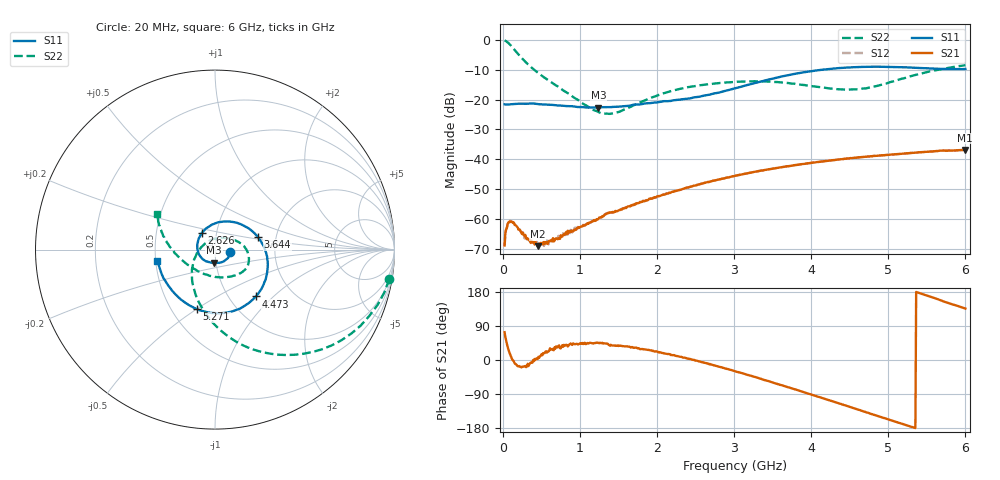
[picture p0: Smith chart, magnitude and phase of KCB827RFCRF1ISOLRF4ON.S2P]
!Agilent Technologies,E5071B,JP1KK00126,A.08.11
!Date: Tue May 06 07:36:09 2014
!Data & Calibration Information:
!Freq	S11:SOLT2(ON)	S21:SOLT2(ON)	S12:SOLT2(ON)	S22:SOLT2(ON)
# Hz S dB R 50
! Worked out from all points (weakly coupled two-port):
!   600 points, 20 MHz to 6 GHz, reference 50 ohm
!   highest |S21| = -36.87 dB at 5.99 GHz (marker M1); lowest = -69.2 dB at 449.3 MHz (marker M2)
!   lowest |S11| = -22.7 dB at 1.238 GHz (marker M3), VSWR 1.16, Z = 48.9 - j7.18 ohm
!   |S11| at or under -10 dB: start of sweep to 4.128 GHz
!   |S22| runs from -24.8 to -0.1 dB; largest |S21 - S12| = 0.00014
!   S11 on the Smith chart (normalised r, x): 20 MHz: 1.18, -0.04; 2.626 GHz: 0.85, +0.16; 3.644 GHz: 1.60, +0.24; 4.473 GHz: 1.32, -0.78; 5.271 GHz: 0.67, -0.50; 6 GHz: 0.51, -0.07
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2e7  -21.58 -10.5  -68.97 73.3  -68.82 78.6  -0.13 -9.6
6.991653e7  -21.63 -7.2  -61.15 27.0  -61.02 27.1  -1.00 -31.7
9.986644e7  -21.55 -9.0  -61.07 10.5  -60.66 10.1  -1.79 -43.1
1.397997e8  -21.46 -11.7  -61.26 -4.1  -61.47 -2.2  -2.99 -56.0
1.996995e8  -21.36 -16.1  -63.61 -16.6  -63.53 -16.1  -4.81 -71.5
2.595993e8  -21.36 -21.1  -64.69 -17.8  -64.78 -18.2  -6.50 -83.3
3.294825e8  -21.34 -28.3  -66.99 -16.2  -67.00 -11.0  -8.29 -94.8
4.492821e8  -21.48 -37.5  -69.18 2.7  -68.50 6.2  -10.91 -111.1
6.09015e8  -21.71 -51.6  -67.40 30.8  -67.71 25.1  -13.84 -129.1
1.018331e9  -22.48 -80.5  -62.51 43.0  -62.68 44.9  -21.03 -177.5
1.237963e9  -22.70 -94.5  -60.03 45.2  -59.72 45.5  -24.18 142.3
1.487546e9  -22.41 -110.6  -57.40 38.2  -57.26 38.6  -24.21 88.1
2.016661e9  -20.85 -157.6  -52.35 21.2  -52.36 20.8  -18.43 26.6
2.625643e9  -18.56 128.7  -47.91 -7.9  -47.88 -7.9  -14.96 -2.6
3.014992e9  -16.17 80.6  -45.54 -30.1  -45.54 -29.7  -14.05 -18.3
3.64394e9  -12.07 16.5  -42.58 -68.6  -42.59 -68.5  -14.30 -43.0
4.013322e9  -10.37 -14.1  -41.19 -91.9  -41.18 -92.2  -15.49 -65.2
4.472554e9  -9.22 -48.9  -39.79 -121.9  -39.83 -122.4  -16.66 -107.0
5.011653e9  -8.99 -87.7  -38.49 -157.6  -38.50 -157.8  -14.22 -163.0
5.271219e9  -9.21 -106.8  -37.96 -174.6  -37.93 -174.7  -12.29 179.0
5.990017e9  -9.72 -167.7  -36.87 136.4  -36.85 136.2  -8.45 148.6
6e9  -9.70 -168.7  -36.88 135.7  -36.87 135.6  -8.43 148.3
